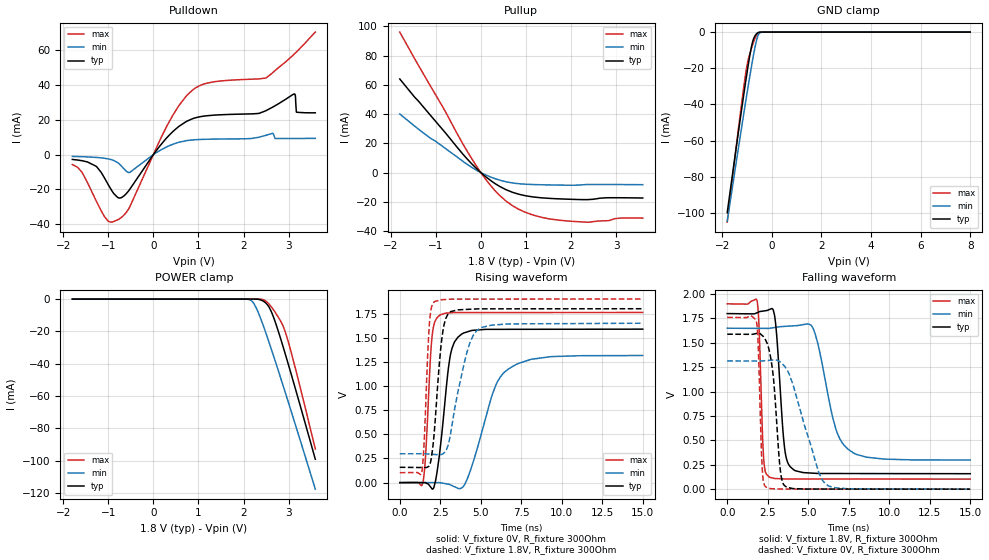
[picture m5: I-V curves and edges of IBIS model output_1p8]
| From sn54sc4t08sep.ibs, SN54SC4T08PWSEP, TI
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|   output_1p8 Model
[Model]   output_1p8
Model_type   3-state
Polarity   Non-Inverting
Vmeas = 0.9
Vref = 0
Cref = 2pF
Rref = 100000
|   typ   min   max
C_comp   5.7pF   5.6pF   6pF
[Voltage Range]   1.8   1.65   1.9
[Temperature Range]   25   125   -40
[Pullup Reference]   1.8   1.65   1.9
[Pulldown Reference]   -0   0   0
[Power Clamp Reference]   1.8   1.65   1.9
[GND Clamp Reference]   0   0   0
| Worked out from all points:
|   slope of the pulldown table from 0 to 0.27 V, typ, clamps not added: 30.4 ohm
|   slope of the pullup table from 0 to 0.27 V, typ, clamps not added: 41 ohm
|   GND clamp passes 1 mA (typ) near -0.62 V on its own axis
|   falling waveform, V_fixture 1.8V, R_fixture 300Ohm: 20-80 % time 400ps typ, 1.07ns min, 210ps max; typ from 1.8 V to 0.159 V
|   rising waveform, V_fixture 0V, R_fixture 300Ohm: 20-80 % time 607ps typ, 1.44ns min, 319ps max; typ from 0 V to 1.59 V
|   rising waveform, V_fixture 1.8V, R_fixture 300Ohm: 20-80 % time 473ps typ, 1ns min, 272ps max; typ from 0.159 V to 1.8 V
|   falling waveform, V_fixture 0V, R_fixture 300Ohm: 20-80 % time 450ps typ, 1.38ns min, 193ps max; typ from 1.59 V to 0 V
[Pulldown]
|   Voltage   I(typ)   I(min)   I(max)
-1.796V   -2.747mA   -1.012mA   -5.67mA
-1.272V   -6.638mA   -1.58mA    -26.32mA
-998.5mV  -17.32mA   -2.453mA   -38.32mA
-778mV    -24.77mA   -4.844mA   -37.27mA
-526mV    -20.04mA   -10.29mA   -30.16mA
282.5mV   9.267mA    4.306mA    15.57mA
755mV     19.36mA    8.123mA    34.36mA
1.165V    22.29mA    8.829mA    40.92mA
2.498V    25.3mA     11.13mA    44.13mA
3.128V    34.89mA    9.29mA     57.91mA
3.17V     24.42mA    9.294mA    58.97mA
3.59V     24.04mA    9.338mA    70.43mA
[GND Clamp]
|   Voltage   I(typ)   I(min)   I(max)
-1.796V   -99.87mA   -104.7mA   -105.2mA
-1.292V   -50.11mA   -59.47mA   -47.76mA
-1.114V   -33.06mA   -43.8mA    -28.76mA
-1.03V    -25.31mA   -36.54mA   -20.87mA
-946mV    -17.88mA   -29.41mA   -14.95mA
-841mV    -9.574mA   -20.75mA   -9.959mA
-778mV    -5.682mA   -15.77mA   -7.246mA
-715mV    -3.091mA   -11.05mA   -4.817mA
-631mV    -1.181mA   -5.509mA   -2.167mA
-536.5mV  -209.2uA   -1.354mA   -383.9uA
-358mV    -660.1nA   -13.32uA   -276.9nA
8V        0A         0A         0A
[Pullup]
|   Voltage   I(typ)   I(min)   I(max)
-1.796V   64mA       40.05mA    96.07mA
-1.188V   41.74mA    25.12mA    62.94mA
-200.5mV  5.964mA    3.551mA    9.465mA
135.5mV   -3.527mA   -1.993mA   -5.757mA
335mV     -7.92mA    -4.387mA   -13.02mA
576.5mV   -11.94mA   -6.412mA   -19.88mA
828.5mV   -14.69mA   -7.579mA   -24.9mA
1.143V    -16.61mA   -8.173mA   -28.89mA
1.752V    -18.01mA   -8.578mA   -32.62mA
2.393V    -18.45mA   -8.164mA   -33.94mA
3.054V    -17.23mA   -8.194mA   -31.21mA
3.59V     -17.39mA   -8.288mA   -31.16mA
[POWER Clamp]
|   Voltage   I(typ)   I(min)   I(max)
-1.796V   -36.89nA   -34.4nA    -37.23nA
2.036V    -24.74nA   -29.44uA   -19.25nA
2.172V    -1.185uA   -1.013mA   -23.19nA
2.236V    -10.71uA   -3.133mA   -120.2nA
2.309V    -102.9uA   -7.226mA   -3.244uA
2.446V    -1.428mA   -17.13mA   -483.2uA
2.55V     -4.388mA   -25.61mA   -2.711mA
2.676V    -12.2mA    -36.24mA   -7.185mA
2.876V    -29.53mA   -53.6mA    -16.76mA
2.96V     -37.4mA    -61.02mA   -23.54mA
3.075V    -48.46mA   -71.3mA    -35.1mA
3.59V     -99.22mA   -117.7mA   -92.85mA
[Ramp]
R_load = 300
|   typ   min   max
dV/dt_r   0.953172/6.04796e-10   0.789366/1.43289e-09   1.05672/3.18602e-10
dV/dt_f   0.984838/3.96886e-10   0.810882/1.06508e-09   1.07817/2.09312e-10
[Falling Waveform]
V_fixture = 1.8V
V_fixture_min = 1.65V
V_fixture_max = 1.9V
R_fixture = 300Ohm
C_fixture = 0F
|   Time   V(typ)   V(min)   V(max)
0s        1.8V       1.65V      1.9V
1.841ns   1.808V     1.648V     1.934V
2.247ns   1.827V     1.648V     319.8mV
2.566ns   1.839V     1.648V     128mV
2.99ns    1.693V     1.659V     109.1mV
3.579ns   376.9mV    1.669V     104.5mV
4.117ns   197mV      1.675V     103.7mV
5.298ns   163.9mV    1.65V      103.6mV
7.444ns   160.2mV    411mV      103.5mV
15ns      158.6mV    298.5mV    103mV
[Rising Waveform]
V_fixture = 0V
V_fixture_min = 0V
V_fixture_max = 0V
R_fixture = 300Ohm
C_fixture = 0F
|   Time   V(typ)   V(min)   V(max)
0s        -1.517uV   -615.1nV   529.4nV
1.424ns   433.4uV    -73.7uV    -3.532mV
1.589ns   -2.101mV   -82.13uV   264.6mV
1.989ns   -63.88mV   -102.7uV   1.506V
2.455ns   297mV      -126.6uV   1.732V
3.127ns   1.321V     -23.24mV   1.757V
3.825ns   1.538V     -53.97mV   1.76V
5.921ns   1.587V     1.005V     1.761V
6.692ns   1.587V     1.174V     1.761V
15ns      1.589V     1.316V     1.761V
[Rising Waveform]
V_fixture = 1.8V
V_fixture_min = 1.65V
V_fixture_max = 1.9V
R_fixture = 300Ohm
C_fixture = 0F
|   Time   V(typ)   V(min)   V(max)
0s        158.6mV    298.5mV    103mV
1.364ns   156.2mV    298.9mV    109.1mV
1.506ns   156mV      298.5mV    424.2mV
1.823ns   178.1mV    295mV      1.631V
2.139ns   540.6mV    291.6mV    1.873V
2.613ns   1.51V      293.9mV    1.893V
3.127ns   1.768V     497.4mV    1.899V
4.153ns   1.793V     1.352V     1.9V
4.972ns   1.799V     1.6V       1.9V
15ns      1.8V       1.65V      1.9V
[Falling Waveform]
|Gnd
V_fixture = 0V
V_fixture_min = 0V
V_fixture_max = 0V
R_fixture = 300Ohm
C_fixture = 0F
|   Time   V(typ)   V(min)   V(max)
0s        1.589V     1.315V     1.761V
1.804ns   1.596V     1.314V     1.715V
1.92ns    1.6V       1.314V     1.438V
2.152ns   1.576V     1.314V     235.7mV
2.369ns   1.529V     1.317V     24.47mV
2.787ns   1.236V     1.323V     4.261mV
3.299ns   165.4mV    1.3V       1.311mV
3.615ns   26.21mV    1.242V     690.4uV
6.197ns   1.295mV    38.38mV    534uV
15ns      -1.604uV   -2.707uV   595.5nV
